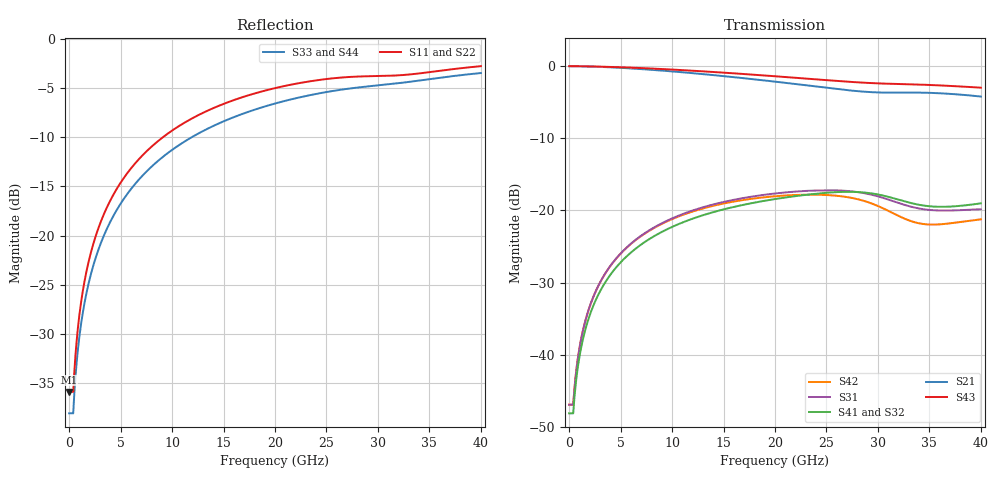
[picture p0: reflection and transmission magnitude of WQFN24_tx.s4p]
! Created Fri Aug 22 07:46:25 2014
# hz S db R 50
! 4 Port Network Data from SP1.SP block
! freq  dbS11  angS11  dbS12  angS12  dbS13  angS13  dbS14  angS14
!  dbS21  angS21  dbS22  angS22  dbS23  angS23  dbS24  angS24
!  dbS31  angS31  dbS32  angS32  dbS33  angS33  dbS34  angS34
!  dbS41  angS41  dbS42  angS42  dbS43  angS43  dbS44  angS44
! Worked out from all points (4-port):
!   4001 points, 1 MHz to 40 GHz, reference 50 ohm
!   strongest paths, dB at 1 MHz, 10 GHz, 20 GHz, 30 GHz, 40 GHz:
!     S43: 0.0, -0.5, -1.4, -2.4, -3.0
!     S21: 0.0, -0.7, -2.2, -3.6, -4.2
!     S41: -48.1, -22.3, -18.4, -17.8, -19.0
!     S31: -46.9, -21.1, -17.7, -18.1, -19.8
!     S32: -48.1, -22.3, -18.5, -17.9, -19.4
!     S42: -46.9, -21.2, -18.0, -19.4, -21.2
!   lowest |S11| = -35.9 dB at 1 MHz (marker M1), VSWR 1.03, Z = 50.1 + j1.61 ohm
!   |S11| at or under -10 dB: start of sweep to 9.123 GHz
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1000000  -35.89 85.9  -0.01 -1.3  -46.93 85.4  -48.12 -95.4
         -0.01 -1.3  -35.89 85.6  -48.12 -95.4  -46.92 85.0
         -46.93 85.4  -48.12 -95.4  -38.07 85.6  -0.01 -1.1
         -48.12 -95.4  -46.92 85.0  -0.01 -1.1  -38.09 85.3
3.71e8  -35.89 85.9  -0.01 -1.3  -46.93 85.4  -48.12 -95.4
        -0.01 -1.3  -35.89 85.6  -48.12 -95.4  -46.92 85.0
        -46.93 85.4  -48.12 -95.4  -38.07 85.6  -0.01 -1.1
        -48.12 -95.4  -46.92 85.0  -0.01 -1.1  -38.09 85.3
1.511e9  -24.57 83.2  -0.04 -5.0  -35.66 80.4  -36.88 -101.6
         -0.04 -5.0  -24.57 82.0  -36.88 -101.5  -35.66 79.1
         -35.66 80.4  -36.88 -101.5  -26.77 83.8  -0.03 -4.3
         -36.88 -101.6  -35.66 79.1  -0.03 -4.3  -26.77 82.5
3.061e9  -18.64 78.7  -0.11 -9.9  -29.83 73.1  -31.06 -110.5
         -0.11 -9.9  -18.65 76.2  -31.06 -110.3  -29.84 70.6
         -29.83 73.1  -31.06 -110.3  -20.83 80.3  -0.07 -8.5
         -31.06 -110.5  -29.84 70.6  -0.07 -8.5  -20.82 77.5
9.681e9  -9.57 61.1  -0.69 -29.5  -21.31 46.2  -22.50 -144.3
         -0.69 -29.5  -9.57 52.9  -22.51 -143.9  -21.41 38.5
         -21.31 46.2  -22.51 -143.9  -11.54 65.4  -0.45 -25.8
         -22.50 -144.3  -21.41 38.5  -0.45 -25.8  -11.55 56.5
2.3261e10  -4.35 32.1  -2.70 -61.8  -17.28 0.9  -17.80 156.7
           -2.70 -61.8  -4.37 12.6  -17.88 157.6  -17.82 -18.0
           -17.28 0.9  -17.88 157.6  -5.76 40.0  -1.75 -56.3
           -17.80 156.7  -17.82 -18.0  -1.75 -56.3  -5.80 18.5
4e10  -2.79 11.9  -4.22 -90.3  -19.83 -26.5  -19.02 107.6
      -4.22 -90.3  -2.69 -20.9  -19.39 109.3  -21.23 -50.3
      -19.83 -26.5  -19.39 109.3  -3.49 19.2  -2.99 -86.7
      -19.02 107.6  -21.23 -50.3  -2.99 -86.7  -3.48 -17.3
